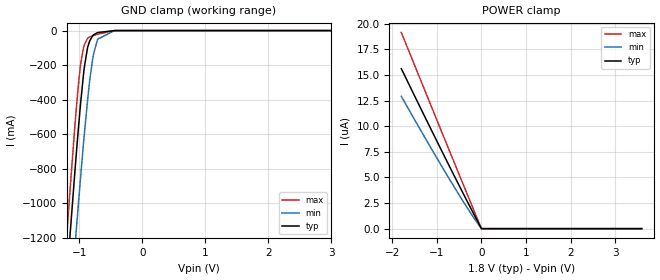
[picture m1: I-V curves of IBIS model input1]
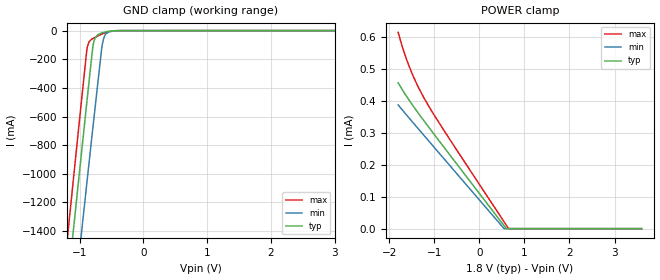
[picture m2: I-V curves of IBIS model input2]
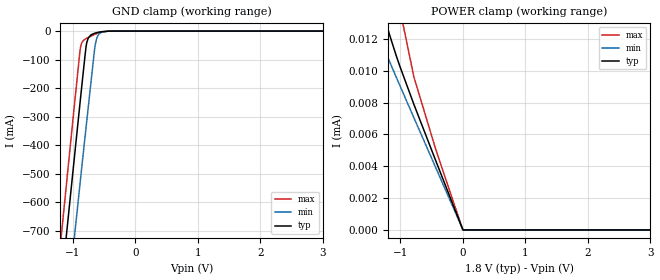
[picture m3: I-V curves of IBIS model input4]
| Texas Instruments Incorporated
| ADS98xx
| 8-Channel, 18-Bit 2/1 MSPS per channel
| With Integrated analog front end
[IBIS Ver]   4.1
[File name]   ads98xx.ibs
[File Rev]   1.0
[Date]   26/12/2023
[Source]
| Texas Instruments Incorporated.
| Analog-eLab Design Center, HPA
| 12500 TI Blvd
| Dallas, TX -75243
[Notes]   Revision History:
| Rev 1.0: 26/12/2023
| - Initial version of the model
| - Model generated from simulations in SPECTRE
| - Model matched to SPICE simulation
| - C_comp although listed in numerical order of value are
|   obtained from varying PVT conditions. For PVT conditions for
|   each specific value refer the buffer description under
|   respective [Model]. IBIS model user is responsible for using
|   appropriate C_comp to simulate for Signal Integrity.
| - Warnings regarding combined Non-monotonicity of various models have been
|   reviewed and considered minor and can be ignored.
[Disclaimer]
| This model is designed as an aid for customers of Texas Instruments.
| TI and its licensors and suppliers make no warranties, either expressed
| or implied, with respect to this  model, including the warranties of
| merchantability or fitness for a particular purpose. The model is
| provided solely on an "as is" basis. The entire risk as to its quality
| and performance is with the customer.
[Copyright]
(C) Copyright 2023 Texas Instruments Incorporated.All rights reserved.
|   ADS9817, ADS9815
[Component]   ADS98xx
[Manufacturer]   TI
[Package]   |56 VQFN
|   typ   min   max
R_pkg   0.07   0.05   0.09
L_pkg   1.1nH   0.8nH   1.4nH
C_pkg   0.18pF   0.15pF   0.21pF
[Pin] signal_name  model_name   R_pin   L_pin   C_pin
1   AIN2P   nc   NA   NA   NA
2   AIN2M   nc   NA   NA   NA
3   AIN3P   nc   NA   NA   NA
4   AIN3M   nc   NA   NA   NA
5   AIN4P   nc   NA   NA   NA
6   AIN4M   nc   NA   NA   NA
7   GND   gnd   NA   NA   NA
8   REFM   nc   NA   NA   NA
9   AIN5P   nc   NA   NA   NA
10   AIN5M   nc   NA   NA   NA
11   AIN6P   nc   NA   NA   NA
12   AIN6M   nc   NA   NA   NA
13   AIN7P   nc   NA   NA   NA
14   AIN7M   nc   NA   NA   NA
15   AVDD_5V   power   NA   NA   NA
16   AIN8P   nc   NA   NA   NA
17   AIN8M   nc   NA   NA   NA
18   REFM   nc   NA   NA   NA
19   REFOUT_2V5   nc   NA   NA   NA
20   NC   nc   NA   NA   NA
21   VDD_1V8   power   NA   NA   NA
22   VDD_1V8   power   NA   NA   NA
23   GND   gnd   NA   NA   NA
24   SPI_EN   input1   NA   NA   NA
25   CSz   input1   NA   NA   NA
26   SCLK   input4   NA   NA   NA
27   SDI   input4   NA   NA   NA
28   SDO   output1   NA   NA   NA
29   IOGND   gnd   NA   NA   NA
30   IOVDD   power   NA   NA   NA
31   RESETz   input4   NA   NA   NA
32   PWDNz   input4   NA   NA   NA
33   DCLKOUT   output2   NA   NA   NA
34   D0   output2   NA   NA   NA
35   D1   output2   NA   NA   NA
36   D2   output2   NA   NA   NA
37   D3   output2   NA   NA   NA
38   NC   nc   NA   NA   NA
39   NC   nc   NA   NA   NA
40   FCLKOUT   output2   NA   NA   NA
41   IOVDD   power   NA   NA   NA
42   IOGND   gnd   NA   NA   NA
43   SMPL_CLKM   input2   NA   NA   NA
44   SMPL_CLKP   input2   NA   NA   NA
45   SMPL_SYNC   input5   NA   NA   NA
46   GND   gnd   NA   NA   NA
47   VDD_1V8   power   NA   NA   NA
48   VDD_1V8   power   NA   NA   NA
49   VDD_1V8   power   NA   NA   NA
50   NC   nc   NA   NA   NA
51   NC   nc   NA   NA   NA
52   REFIO   nc   NA   NA   NA
53   REFM   nc   NA   NA   NA
54   AIN1P   nc   NA   NA   NA
55   AIN1M   nc   NA   NA   NA
56   AVDD_5V   power   NA   NA   NA
| Models and submodels in the file (6): input1 (Input), input2 (Input), input4 (Input), input5 (Input), output1 (3-state), output2 (Output)
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|   input1 Model
[Model]   input1
Model_type   Input
Vinl = 0.54
Vinh = 1.26
|   typ   min   max
C_comp   0.672pF   0.636pF   0.697pF
[Voltage Range]   1.8   1.75   1.85
[Temperature Range]   27   125   -40
[Power Clamp Reference]   1.8   1.75   1.85
[GND Clamp Reference]   0   0   0
[GND Clamp]
|   Voltage   I(typ)   I(min)   I(max)
-1.8V     -4.321A    -4.211A    -4.387A
-1.195V   -1.418A    -1.849A    -1.162A
-1.147V   -1.178A    -1.615A    -916mA
-1.044V   -693.2mA   -1.134A    -431.7mA
-984.6mV  -438.2mA   -867.3mA   -208.3mA
-936mV    -259.3mA   -660.5mA   -102.1mA
-871.2mV  -101.4mA   -409.6mA   -46.07mA
-838.8mV  -63.14mA   -300.5mA   -37.3mA
-774mV    -23.82mA   -134.1mA   -29.01mA
-709.2mV  -11.34mA   -50.08mA   -20.86mA
-444.6mV  -226.7uA   -207uA     -338.8uA
3.6V      0A         0A         0A
[POWER Clamp]
|   Voltage   I(typ)   I(min)   I(max)
-1.8V     15.62uA    12.93uA    19.16uA
-1.222V   10.49uA    8.533uA    12.96uA
-720mV    6.094uA    4.84uA     7.608uA
-309.6mV  2.579uA    1.973uA    3.258uA
-1.8mV    10.88nA    7.532nA    14.89nA
3.6V      0A         0A         0A
|   input2 Model
[Model]   input2
Model_type   Input
Vinl = 0.54
Vinh = 1.26
|   typ   min   max
C_comp   1.84pF   1.72pF   2.03pF
[Voltage Range]   1.8   1.75   1.85
[Temperature Range]   27   125   -40
[Power Clamp Reference]   1.8   1.75   1.85
[GND Clamp Reference]   0   0   0
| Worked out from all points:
|   GND clamp passes 1 mA (typ) near -0.44 V on its own axis
[GND Clamp]
|   Voltage   I(typ)   I(min)   I(max)
-1.8V     -4.415A    -4.911A    -4.109A
-1.33V    -2.396A    -2.926A    -2.058A
-1.12V    -1.494A    -2.04A     -1.141A
-1.055V   -1.218A    -1.769A    -859.4mA
-1.006V   -1.011A    -1.566A    -648.9mA
-882mV    -486.1mA   -1.051A    -125.9mA
-784.8mV  -96.7mA    -656.1mA   -54.09mA
-709.2mV  -27.49mA   -351.2mA   -36.6mA
-649.8mV  -16.05mA   -116.8mA   -24.29mA
-622.8mV  -12.53mA   -57.25mA   -19.32mA
-536.4mV  -4.706mA   -7.688mA   -7.279mA
3.6V      0A         0A         0A
[POWER Clamp]
|   Voltage   I(typ)   I(min)   I(max)
-1.8V     456.5uA    387.1uA    614uA
-1.681V   428.7uA    366.9uA    557.6uA
-1.611V   413.4uA    355.2uA    528.6uA
-1.508V   392.1uA    338.1uA    491.1uA
-1.336V   358uA      309.5uA    438uA
-1.179V   328.2uA    283.7uA    397.1uA
-790.2mV  255.9uA    219.8uA    308.4uA
549mV     9.364uA    174.3nA    21.56uA
597.6mV   426.3nA    0A         11.18uA
646.2mV   0A         0A         795.4nA
3.6V      0A         0A         0A
|   input4 Model
[Model]   input4
Model_type   Input
Vinl = 0.54
Vinh = 1.26
|   typ   min   max
C_comp   0.383pF   0.369pF   0.397pF
[Voltage Range]   1.8   1.75   1.85
[Temperature Range]   27   125   -40
[Power Clamp Reference]   1.8   1.75   1.85
[GND Clamp Reference]   0   0   0
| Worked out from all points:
|   GND clamp passes 1 mA (typ) near -0.48 V on its own axis
[GND Clamp]
|   Voltage   I(typ)   I(min)   I(max)
-1.8V     -2.211A    -2.457A    -2.059A
-1.082V   -666.2mA   -940.9mA   -487.6mA
-1.001V   -493.3mA   -771.4mA   -311.3mA
-882mV    -241.6mA   -524.9mA   -61.23mA
-855mV    -185.2mA   -469.4mA   -40.08mA
-784.8mV  -47.19mA   -326.8mA   -25.75mA
-757.8mV  -25.6mA    -272.2mA   -22.63mA
-709.2mV  -12.91mA   -174.2mA   -17.31mA
-649.8mV  -7.402mA   -57.4mA    -11.39mA
-622.8mV  -5.724mA   -27.78mA   -9.01mA
-536.4mV  -2.04mA    -3.437mA   -3.272mA
3.6V      0A         0A         0A
[POWER Clamp]
|   Voltage   I(typ)   I(min)   I(max)
-1.8V     29.43uA    17.45uA    104.2uA
-1.379V   15.38uA    12.52uA    31.27uA
-1.26V    13.44uA    11.38uA    23.11uA
-1.179V   12.32uA    10.63uA    19.25uA
-1.012V   10.31uA    9.097uA    13.93uA
-784.8mV  7.891uA    7.052uA    9.614uA
-444.6mV  4.447uA    3.999uA    5.187uA
-1.8mV    16nA       28.77nA    19.1nA
3.6V      0A         0A         0A
